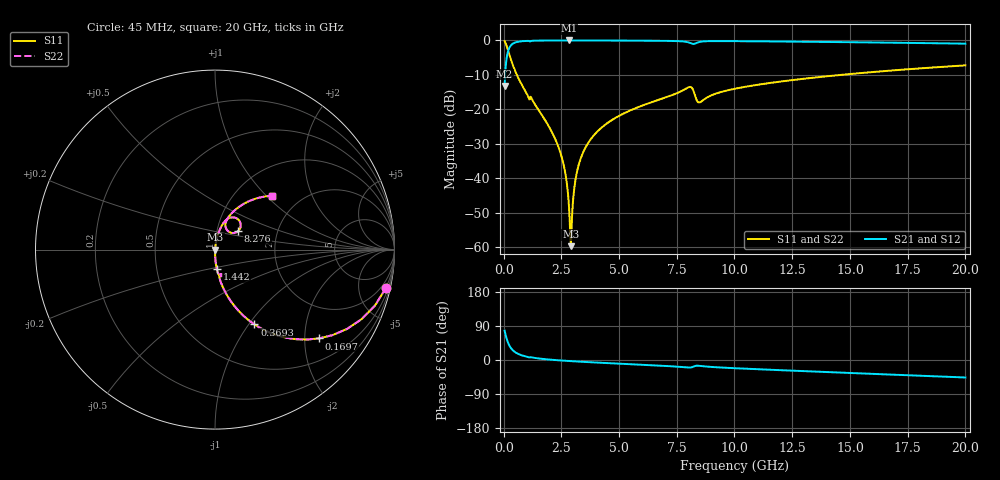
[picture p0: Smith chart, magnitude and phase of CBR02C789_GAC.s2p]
! S-parameter model data by Modelithics Inc.  support@modelithics.com 813-866-6335  Tampa FL USA
! S-Parameter data specifications:
! Substrate: 20-mil Rogers 4350B, substrate thickness, H=0.508mm, Dielectric constant, Er=3.75
! PCB Mounting Pad Footprint: Pad width, PadW=0.32mm , Pad length, PadL=0.37mm , Pad gap, PadG (edge-to-edge)=0.19mm , Reference planes=0.93mm apart
#  GHz  S  MA  R 50
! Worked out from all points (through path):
!   801 points, 45 MHz to 20 GHz, reference 50 ohm
!   highest |S21| = -0.01 dB at 2.839 GHz (marker M1); lowest = -13.2 dB at 45 MHz (marker M2)
!   group delay of S21, straight-line fit = 8.08 ps
!   lowest |S11| = -59.6 dB at 2.914 GHz (marker M3), VSWR 1.00, Z = 50.1 + j0.0103 ohm
!   |S11| at or under -10 dB: 576.8 MHz to 14.59 GHz (14.01 GHz wide, 185 % of centre)
!   |S22| runs from -59.6 to -0.2 dB; largest |S21 - S12| = 0
!   S11 on the Smith chart (normalised r, x): 45 MHz: 0.99, -8.89; 169.7 MHz: 0.99, -2.35; 369.3 MHz: 0.99, -1.07; 1.442 GHz: 1.00, -0.21; 8.276 GHz: 1.26, +0.27; 20 GHz: 1.45, +1.07
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0.045  0.9758 -12.7  0.2188 77.3  0.2188 77.3  0.9758 -12.7
0.169719  0.7624 -40.5  0.6467 49.5  0.6467 49.5  0.7624 -40.5
0.369269  0.4711 -62.2  0.8814 27.7  0.8814 27.7  0.4711 -62.2
0.718481  0.2524 -75.9  0.9667 13.9  0.9667 13.9  0.2524 -75.9
1.44185  0.1069 -84.8  0.9932 4.7  0.9932 4.7  0.1069 -84.8
2.464544  0.02339 -88.8  0.9987 -1.2  0.9987 -1.2  0.02339 -88.8
2.689037  0.01113 -86.9  0.9989 -2.1  0.9989 -2.1  0.01113 -86.9
2.8387  0.003635 -76.4  0.9989 -2.7  0.9989 -2.7  0.003635 -76.4
2.913531  0.001042 5.7  0.9989 -3.0  0.9989 -3.0  0.001042 5.7
2.988363  0.003855 71.1  0.9989 -3.3  0.9989 -3.3  0.003855 71.1
3.138025  0.01063 80.5  0.9988 -3.8  0.9988 -3.8  0.01063 80.5
3.387462  0.02143 82.4  0.9986 -4.7  0.9986 -4.7  0.02143 82.4
3.811506  0.03843 82.2  0.9981 -6.1  0.9981 -6.1  0.03843 82.2
4.460044  0.06214 80.8  0.9968 -8.1  0.9968 -8.1  0.06214 80.8
6.704981  0.1374 74.3  0.9881 -14.7  0.9881 -14.7  0.1374 74.3
8.027  0.2103 57.3  0.9323 -20.0  0.9323 -20.0  0.2103 57.3
8.276438  0.1651 38.7  0.8956 -16.2  0.8956 -16.2  0.1651 38.7
8.500931  0.1265 56.2  0.953 -15.5  0.953 -15.5  0.1265 56.2
10.0225  0.1996 67.2  0.976 -21.7  0.976 -21.7  0.1996 67.2
13.36496  0.2872 59.3  0.9553 -30.3  0.9553 -30.3  0.2872 59.3
16.68248  0.3638 51.3  0.9288 -38.3  0.9288 -38.3  0.3638 51.3
20  0.4351 43.5  0.8976 -46.2  0.8976 -46.2  0.4351 43.5
